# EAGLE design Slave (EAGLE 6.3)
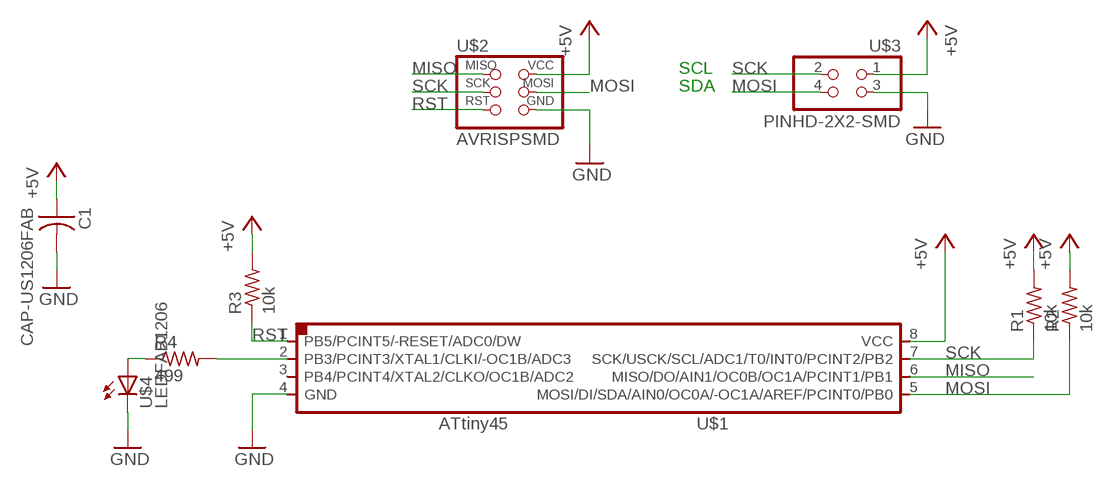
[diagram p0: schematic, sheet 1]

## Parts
C1  CAP-US1206FAB  [C1206FAB]
R1  10k  RES-US1206FAB  [R1206FAB]
R2  10k  RES-US1206FAB  [R1206FAB]
R3  10k  RES-US1206FAB  [R1206FAB]
R4  499  RES-US1206FAB  [R1206FAB]
U$1  ATTINY45SI  [SOIC8]
U$2  AVRISPSMD  [2X03SMD]
U$3  PINHD-2X2-SMD  [2X02SMD]
U$4  LEDFAB1206  [LED1206FAB]

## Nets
+5V: C1.1 R1.2 R2.2 R3.2 U$1.8(VCC) U$2.2(VCC) U$3.1
GND: C1.2 U$1.4(GND) U$2.6(GND) U$3.3 U$4.2(C)
MISO: U$1.6(MISO/DO/AIN1/OC0B/OC1A/PCINT1/PB1) U$2.1(MISO)
MOSI: R2.1 U$1.5(MOSI/DI/SDA/AIN0/OC0A/-OC1A/AREF/PCINT0/PB0) U$2.4(MOSI) U$3.4
N$1: R4.1 U$4.1(A)
N$2: R4.2 U$1.2(PB3/PCINT3/XTAL1/CLKI/-OC1B/ADC3)
RST: R3.1 U$1.1(PB5/PCINT5/-RESET/ADC0/DW) U$2.5(RST)
SCK: R1.1 U$1.7(SCK/USCK/SCL/ADC1/T0/INT0/PCINT2/PB2) U$2.3(SCK) U$3.2
Unconnected: U$1.3(PB4/PCINT4/XTAL2/CLKO/OC1B/ADC2)

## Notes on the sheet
- SCL
- SDA

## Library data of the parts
C1 = fab:CAP-US
R1-R4 = fab:RES-US: Resistor (US Symbol)
U$1 = fab:ATTINY45
U$2 = fab:AVRISP
U$3 = fab:PINHD-2X2-SMD
U$4 = fab:LED: LED

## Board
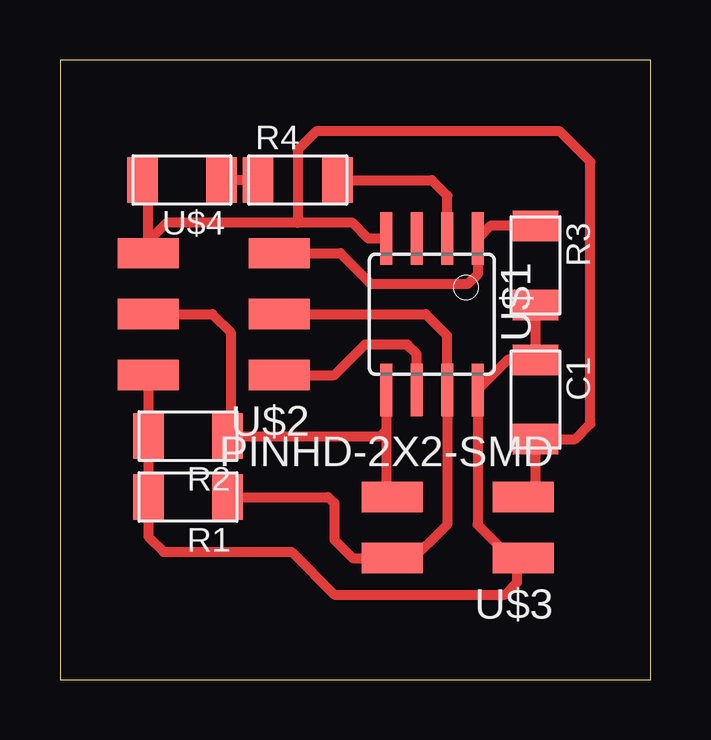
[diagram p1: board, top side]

Size 24.62 x 25.83 mm. Coordinates in mm from the lower left corner, seen from the top.
Outline: 0,0 24.62,0 24.62,25.83 0,25.83 0,0
Copper layers (1*16): Top 0.035mm / dielectric 1.5mm / Bottom 0.035mm
Design rules "default": minimum track width 10mil, minimum drill 24mil, track to track 8mil, track to pad 8mil, pad to pad 8mil, via to via 8mil, smd to smd 8mil, copper to edge 40mil, drill to drill 8mil, minimum pad ring 10mil, minimum via ring 8mil, stop-mask expansion 4mil, vias tented up to drill 0mil, thermal gap 10mil

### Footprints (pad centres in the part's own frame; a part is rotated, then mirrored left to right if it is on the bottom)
C1206FAB = smd 1.27 x 1.905: 1 -1.651,0; 2 1.651,0
R1206FAB = smd 1.27 x 1.905: 1 -1.651,0; 2 1.651,0
SOIC8 = smd 0.5 x 2.2: 1 -1.905,-3.154; 2 -0.645,-3.154; 3 0.625,-3.154; 4 1.895,-3.154; 5 1.905,3.154; 6 0.635,3.154; 7 -0.635,3.154; 8 -1.905,3.154
2X03SMD = smd 2.54 x 1.27: 1 -2.54,2.54; 2 2.92,2.54; 3 -2.54,0; 4 2.92,0; 5 -2.54,-2.54; 6 2.92,-2.54
2X02SMD = smd 2.54 x 1.27: 1 -2.54,1.27; 2 2.92,1.27; 3 -2.54,-1.27; 4 2.92,-1.27
LED1206FAB = smd 1.27 x 1.905: 1 -1.651,0; 2 1.651,0

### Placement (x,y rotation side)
C1  19.81,11.68 270 top
R1  5.33,7.62 180 top
R2  5.33,10.16 180 top
R3  19.81,17.27 270 top
R4  9.91,20.83 0 top
U$1  15.49,15.24 180 top
U$2  6.6,15.24 180 top
U$3  16.76,6.35 180 top
U$4  5.08,20.83 180 top

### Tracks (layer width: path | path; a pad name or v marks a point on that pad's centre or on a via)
+5V
  Top 0.406: U$2.2 R2.2 R1.2 3.68,5.97 4.32,5.33 9.65,5.33 11.43,3.56 18.54,3.56 19.05,4.06 19.05,4.83 U$3.1 18.8,5.08 17.4,6.48 U$1.8 18.65,13.34 C1.1 R3.2
GND
  Top 0.406: U$2.6 3.68,18.29 | 3.68,18.29 3.68,20.57 U$4.2 | U$1.4 12.85,18.39 12.19,19.05 9.91,19.05 | 9.91,19.05 4.45,19.05 3.68,18.29 | U$3.3 19.81,8.13 C1.2 21.46,10.03 22.1,10.67 22.1,21.59 20.83,22.86 10.67,22.86 9.91,22.1 9.91,19.05
MISO
  Top 0.406: U$2.1 11.43,12.7 12.7,13.97 14.48,13.97 14.86,13.59 U$1.6
MOSI
  Top 0.406: U$1.5 13.59,10.41 | 13.59,10.41 13.59,7.88 U$3.4 | U$2.4 6.35,15.24 7.11,14.48 7.11,10.29 R2.1 13.34,10.16 13.59,10.41
N$1
  Top 0.406: R4.1 U$4.1
N$2
  Top 0.406: R4.2 15.49,20.83 16.14,20.18 U$1.2
RST
  Top 0.406: U$2.5 11.68,17.78 12.95,16.51 17.02,16.51 17.4,16.89 U$1.1 17.93,18.92 R3.1
SCK
  Top 0.406: U$2.3 15.24,15.24 16.13,14.35 U$1.7 16.13,6.48 14.48,4.83 14.1,4.83 U$3.2 12.19,5.08 11.43,5.84 11.43,7.37 11.18,7.62 R1.1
